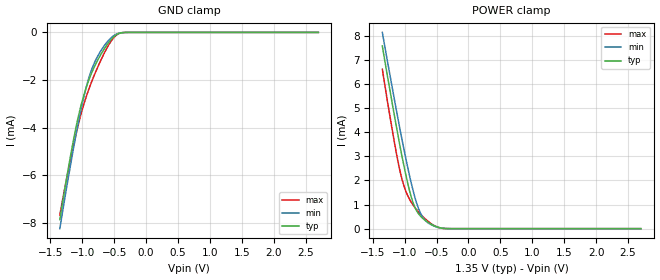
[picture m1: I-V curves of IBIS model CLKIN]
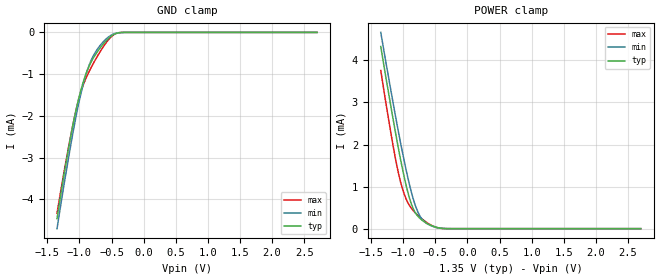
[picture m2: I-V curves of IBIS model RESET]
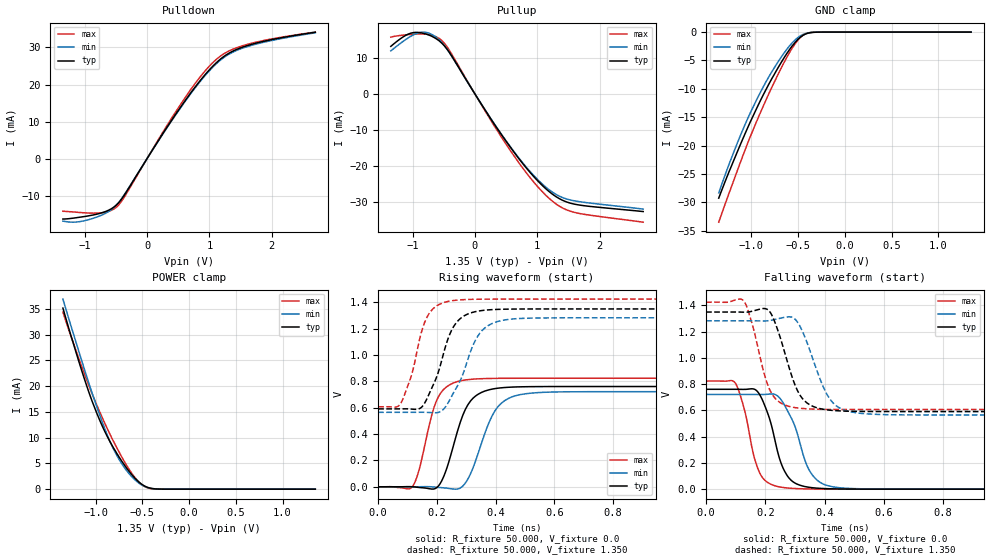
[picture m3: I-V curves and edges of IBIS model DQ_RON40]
| This Model is valid for Temperature Range -40C<=Tc<=95C
| Valid for DDR3-1600/1866 operation
| Part Number   VDD/VDDQ   Architecture   Package
| SCB13H8G162DF_DIE   1.35V/1.35V   512Mx8   Bare Die
[IBIS ver]  5.1
[File name] scb13h8g162df_die.ibs
[File Rev]  1.10
[Date]   2024-08-01
[Source]   Simulation of a silicon level SPICE model
[Notes]   Revision History:
   Rev 1.00: 2024-05-20
   - Initial release
   Rev 1.10: 2024-08-01
   - add bare die model
[Disclaimer]  The IBIS models are for modeling purpose only and are
   subject to change without any notice. UniIC is not
   responsible for any problems the models may cause.
[Copyright] Copyright 2024 UniIC Semiconductors Corp. All rights reserved
| COMPONENT: SCB13H8G162DF_DIE (Bare Die)
[Component]   SCB13H8G162DF_DIE
[Manufacturer]  UniIC Semiconductors Corp.
[Package]
|   typ   min   max
R_pkg   0.001m   0.001m   0.001m
L_pkg   0.001nH   0.001nH   0.001nH
C_pkg   0.001pF   0.001pF   0.001pF
[Pin]   signal_name   model_name   R_pin   L_pin   C_pin
1   VSS   GND
2   VDDP   POWER
3   VDD   POWER
4   RESETB   RESET
5   VDD   POWER
6   A13   INPUT
7   A9   INPUT
8   A7   INPUT
9   A2   INPUT
10   A5   INPUT
11   A0   INPUT
12   A3   INPUT
13   BA2   INPUT
14   BA0   INPUT
15   VSS   GND
16   VDD   POWER
17   WEB   INPUT
18   CSB   INPUT
19   CASB   INPUT
20   ODT   ODT
21   RASB   INPUT
22   VDD   POWER
23   VSS   GND
24   VREFDQ   POWER
25   VSS   GND
26   DQL7   DQ
27   VDDQ   POWER
28   VSS   GND
29   DQL5   DQ
30   VDDQ   POWER
31   DQL3   DQ
32   VSS   GND
33   DQL1   DQ
34   VSS   GND
35   DML   DM
36   VSS   GND
37   VDD   POWER
38   VSS   GND
39   VSS   GND
40   VDD   POWER
41   VSS   GND
42   A14   INPUT
43   A11   INPUT
44   A8   INPUT
45   A1   INPUT
46   A6   INPUT
47   A4   INPUT
48   VSS   GND
49   VDD   POWER
50   A12   INPUT
51   A15   INPUT
52   BA1   INPUT
53   ZQ   INPUT
54   VREFCA   POWER
55   A10   INPUT
56   CKE   INPUT
57   CKB   CLKIN
58   CK   CLKIN
59   VSS   GND
60   VDD   POWER
61   DQL4   DQ
62   VDDQ   POWER
63   DQL6   DQ
64   VSS   GND
65   DQSLB   DQS
66   DQSL   DQS
67   DQL2   DQ
68   VDDQ   POWER
69   DQL0   DQ
70   VDDQ   POWER
71   VDD   POWER
72   VDDQ   POWER
|**********************DIFF PIN*********************************************
[Diff_pin]   inv_pin   vdiff   tdelay_typ   tdelay_min   tdelay_max
   58   57   0.320V   0ns   NA   NA
   66   65   0.320V   0ns   NA   NA
|   Model Selector
[Model Selector] DQ
DQ_RON34   DQ  With 34ohm driving & Without ODT
DQ_RON40   DQ  With 40ohm driving & Without ODT
DQ_ODTOFF   DQ  Input with ODT OFF
DQ_ODT20   DQ  Input with 20ohm ODT
DQ_ODT30   DQ  Input with 30ohm ODT
DQ_ODT40   DQ  Input with 40ohm ODT
DQ_ODT60   DQ  Input with 60ohm ODT
DQ_ODT120   DQ  Input with 120ohm ODT
[Model Selector] DQS
DQS_RON34   DQS with 34ohm driving & Without ODT
DQS_RON40   DQS with 40ohm driving & Without ODT
DQS_ODTOFF   DQS Input with ODT OFF
DQS_ODT20   DQS Input with 20ohm ODT
DQS_ODT30   DQS Input with 30ohm ODT
DQS_ODT40   DQS Input with 40ohm ODT
DQS_ODT60   DQS Input with 60ohm ODT
DQS_ODT120   DQS Input with 120ohm ODT
[Model Selector] DM
DM_ODTOFF   DM Input with ODT OFF
DM_ODT20   DM Input with 20ohm ODT
DM_ODT30   DM Input with 30ohm ODT
DM_ODT40   DM Input with 40ohm ODT
DM_ODT60   DM Input with 60ohm ODT
DM_ODT120   DM Input with 120ohm ODT
| Models and submodels in the file (41): CLKIN (Input), INPUT (Input), RESET (Input), ODT (Input), DQ_RON34 (I/O), DQ_RON40 (I/O), DQ_ODTOFF (Input), DQ_ODT20 (Input), DQ_ODT30 (Input), DQ_ODT40 (Input), DQ_ODT60 (Input), DQ_ODT120 (Input), DQS_RON34 (I/O), DQS_RON40 (I/O), DQS_ODTOFF (Input), DQS_ODT20 (Input), DQS_ODT30 (Input), DQS_ODT40 (Input), DQS_ODT60 (Input), DQS_ODT120 (Input), DM_ODTOFF (Input), DM_ODT20 (Input), DM_ODT30 (Input), DM_ODT40 (Input), DM_ODT60 (Input), DM_ODT120 (Input), DQ_20ohm_ODT (Dynamic_clamp), DQ_30ohm_ODT (Dynamic_clamp), DQ_40ohm_ODT (Dynamic_clamp), DQ_60ohm_ODT (Dynamic_clamp), DQ_120ohm_ODT (Dynamic_clamp), DQS_20ohm_ODT (Dynamic_clamp), DQS_30ohm_ODT (Dynamic_clamp), DQS_40ohm_ODT (Dynamic_clamp), DQS_60ohm_ODT (Dynamic_clamp), DQS_120ohm_ODT (Dynamic_clamp), DM_20ohm_ODT (Dynamic_clamp), DM_30ohm_ODT (Dynamic_clamp), DM_40ohm_ODT (Dynamic_clamp), DM_60ohm_ODT (Dynamic_clamp), DM_120ohm_ODT (Dynamic_clamp)
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|   Model CLKIN
[Model] CLKIN
Model_type Input
Polarity   Non-Inverting
Enable   Active-High
Vinl =  0.550V
Vinh =  0.800V
C_comp   0.645pF   0.638pF   0.647pF
C_comp_power_clamp   0.143pF   0.139pF   0.145pF
C_comp_gnd_clamp   0.502pF   0.500pF   0.502pF
[Temperature Range]   45.000   95.000   -40.000
[Voltage Range]   1.350V   1.283V   1.425V
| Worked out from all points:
|   GND clamp passes 1 mA (typ) near -0.72 V on its own axis
|   POWER clamp passes 1 mA (typ) near -0.86 V on its own axis
[GND_clamp]
|Voltage   I(typ)   I(min)   I(max)
-1.35V    -7.873mA   -8.253mA   -7.683mA
-1.238V   -6.036mA   -6.436mA   -6.079mA
-1.125V   -4.374mA   -4.714mA   -4.633mA
-1.013V   -3.021mA   -3.17mA    -3.382mA
-928mV    -2.251mA   -2.219mA   -2.636mA
-844mV    -1.655mA   -1.511mA   -2.025mA
-759mV    -1.181mA   -1.013mA   -1.48mA
-619mV    -551.5uA   -436.8uA   -691.9uA
-506mV    -188.5uA   -137.9uA   -224uA
-422mV    -44.43uA   -32.03uA   -42.35uA
-338mV    -5.118uA   -4.402uA   -2.782uA
2.7V      0A         0A         0A
[POWER_clamp]
|Voltage   I(typ)   I(min)   I(max)
-1.35V    7.585mA    8.149mA    6.621mA
-1.153V   4.58mA     5.252mA    3.47mA
-1.097V   3.766mA    4.457mA    2.689mA
-1.041V   2.988mA    3.686mA    2.041mA
-984mV    2.262mA    2.946mA    1.57mA
-928mV    1.619mA    2.251mA    1.24mA
-844mV    908.9uA    1.339mA    892.5uA
-759mV    541.8uA    679.8uA    624.6uA
-647mV    285.5uA    268.6uA    333.7uA
-506mV    86.29uA    73.86uA    85.78uA
-366mV    7.504uA    7.144uA    3.873uA
2.7V      0A         0A         0A
|   Model RESET
[Model] RESET
Model_type Input
Polarity   Non-Inverting
Enable   Active-High
Vinl =  0.270V
Vinh =  1.080V
C_comp   0.551pF   0.542pF   0.555pF
C_comp_power_clamp   0.114pF   0.109pF   0.116pF
C_comp_gnd_clamp   0.437pF   0.433pF   0.439pF
[Temperature Range]   45.000   95.000   -40.000
[Voltage Range]   1.350V   1.283V   1.425V
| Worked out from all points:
|   GND clamp passes 1 mA (typ) near -0.90 V on its own axis
|   POWER clamp passes 1 mA (typ) near -0.95 V on its own axis
[GND_clamp]
|Voltage   I(typ)   I(min)   I(max)
-1.35V    -4.459mA   -4.699mA   -4.332mA
-1.238V   -3.374mA   -3.617mA   -3.314mA
-1.097V   -2.175mA   -2.364mA   -2.167mA
-1.013V   -1.587mA   -1.704mA   -1.607mA
-928mV    -1.122mA   -1.16mA    -1.204mA
-872mV    -885.7uA   -877.9uA   -1.006mA
-788mV    -622.5uA   -570.5uA   -752.1uA
-675mV    -364.9uA   -305.9uA   -453.3uA
-563mV    -165.4uA   -128.1uA   -202.9uA
-450mV    -38.09uA   -27.42uA   -40.32uA
-338mV    -2.553uA   -2.201uA   -1.39uA
2.7V      0A         0A         0A
[POWER_clamp]
|Voltage   I(typ)   I(min)   I(max)
-1.35V    4.331mA    4.667mA    3.761mA
-1.266V   3.557mA    3.918mA    2.946mA
-1.153V   2.561mA    2.949mA    1.928mA
-1.069V   1.859mA    2.255mA    1.281mA
-1.012V   1.425mA    1.815mA    950.8uA
-928mV    862.1uA    1.21mA     617uA
-844mV    472.4uA    705.3uA    428.3uA
-759mV    272.3uA    354.4uA    298.8uA
-647mV    139.8uA    137.3uA    161uA
-506mV    42.4uA     36.88uA    42.07uA
-366mV    3.748uA    3.583uA    1.942uA
2.7V      0A         0A         0A
|   Model DQ_RON40
[Model] DQ_RON40
Model_type I/O
Polarity   Non-Inverting
Enable   Active-High
Vinl =  0.545V
Vinh =  0.805V
Vmeas =  0.675V
Cref =  0.0F
Rref =  50.000
Vref =  0.675V
C_comp   0.962pF   0.943pF   0.974pF
C_comp_pullup   0.232pF   0.222pF   0.238pF
C_comp_pulldown   0.730pF   0.721pF   0.736pF
[Temperature Range]   45.000   95.000   -40.000
[Voltage Range]   1.350V   1.283V   1.425V
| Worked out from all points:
|   slope of the pulldown table from 0 to 0.203 V, typ, clamps not added: 37.6 ohm
|   slope of the pullup table from 0 to 0.203 V, typ, clamps not added: 36.9 ohm
|   GND clamp passes 1 mA (typ) near -0.48 V on its own axis
|   POWER clamp passes 1 mA (typ) near -0.51 V on its own axis
|   rising waveform, R_fixture 50.000, V_fixture 0.0: 20-80 % time 66.8ps typ, 75.1ps min, 56.5ps max; typ from 0 V to 0.761 V
|   rising waveform, R_fixture 50.000, V_fixture 1.350: 20-80 % time 71.2ps typ, 82.6ps min, 59.3ps max; typ from 0.591 V to 1.35 V
|   falling waveform, R_fixture 50.000, V_fixture 0.0: 20-80 % time 58.8ps typ, 68.9ps min, 50.6ps max; typ from 0.761 V to 0 V
|   falling waveform, R_fixture 50.000, V_fixture 1.350: 20-80 % time 66.4ps typ, 74.8ps min, 57.3ps max; typ from 1.35 V to 0.591 V
[Pulldown]
|Voltage   I(typ)   I(min)   I(max)
-1.35V    -16.29mA   -16.85mA   -14.19mA
-1.145V   -15.96mA   -17.11mA   -14.43mA
-900mV    -15.31mA   -16.28mA   -14.69mA
-655mV    -14.19mA   -14.64mA   -14.39mA
-491mV    -12.5mA    -12.53mA   -13.09mA
-368mV    -9.933mA   -9.803mA   -10.47mA
286mV     7.58mA     7.47mA     8.003mA
695mV     17.6mA     17.38mA    18.5mA
982mV     23.62mA    23.37mA    24.62mA
1.227V    27.49mA    27.22mA    28.23mA
1.718V    31.02mA    30.76mA    31.29mA
2.7V      34.1mA     33.95mA    34.14mA
[Pullup]
|Voltage   I(typ)   I(min)   I(max)
-1.35V    13.16mA    11.91mA    15.72mA
-1.105V   16.28mA    15.14mA    16.36mA
-900mV    17.01mA    16.95mA    16.6mA
-736mV    16.29mA    16.81mA    16.44mA
-573mV    14.68mA    14.95mA    15.34mA
-409mV    11.44mA    11.45mA    12.06mA
245mV     -6.628mA   -6.587mA   -7.019mA
695mV     -17.68mA   -17.5mA    -18.8mA
1.023V    -24.32mA   -23.97mA   -25.96mA
1.309V    -28.49mA   -27.86mA   -30.52mA
1.636V    -30.61mA   -29.69mA   -32.92mA
2.7V      -32.53mA   -31.85mA   -35.47mA
[GND_clamp]
|Voltage   I(typ)   I(min)   I(max)
-1.35V    -29.26mA   -28.34mA   -33.49mA
-1.238V   -24.53mA   -23.21mA   -28.3mA
-1.097V   -18.99mA   -17.39mA   -22.02mA
-1.013V   -15.85mA   -14.25mA   -18.44mA
-872mV    -11.01mA   -9.597mA   -12.98mA
-731mV    -6.729mA   -5.642mA   -7.982mA
-619mV    -3.711mA   -2.975mA   -4.366mA
-534mV    -1.839mA   -1.403mA   -2.088mA
-450mV    -579.7uA   -428.9uA   -569.3uA
-394mV    -185.5uA   -144.2uA   -144.2uA
-281mV    -9.318uA   -9.811uA   -3.103uA
1.35V     0A         0A         0A
[POWER_clamp]
|Voltage   I(typ)   I(min)   I(max)
-1.35V    35.16mA    36.91mA    34.39mA
-1.181V   24.89mA    26.83mA    25.44mA
-1.069V   18.67mA    20.39mA    19.96mA
-956mV    13.38mA    14.37mA    15mA
-872mV    10.11mA    10.36mA    11.63mA
-787mV    7.358mA    7.025mA    8.526mA
-703mV    4.977mA    4.465mA    5.69mA
-619mV    2.933mA    2.534mA    3.219mA
-534mV    1.338mA    1.137mA    1.316mA
-450mV    385.5uA    342uA      284.3uA
-366mV    62.9uA     66.43uA    27.04uA
1.35V     0A         0A         9.135nA
[Ramp]
| variable   typ   min   max
dV/dt_r   0.457/67.068p   0.433/75.437p   0.494/56.454p
dV/dt_f   0.455/66.331p   0.431/74.640p   0.491/58.220p
R_load = 50.000
[Rising Waveform]
R_fixture= 50.000
V_fixture= 0.0
V_fixture_min= 0.0
V_fixture_max= 0.0
|time   V(typ)   V(min)   V(max)
0s        104.4nV    279.9nV    10.03uV
119ps     -364.1uV   -73.9uV    8.881mV
203ps     464.6uV    -4.308mV   673.4mV
232ps     129.5mV    -10.12mV   756.8mV
280ps     492mV      -8.598mV   804mV
325ps     676mV      154.5mV    817.3mV
378ps     736.2mV    489.8mV    822.1mV
411ps     749.3mV    615.4mV    823.2mV
543ps     760.4mV    714.7mV    824mV
5ns       761.1mV    722mV      824mV
[Rising Waveform]
R_fixture= 50.000
V_fixture= 1.350
V_fixture_min= 1.283
V_fixture_max= 1.425
|time   V(typ)   V(min)   V(max)
0s        591.3mV    565.2mV    607mV
79ps      591.3mV    565.2mV    642mV
114ps     589.6mV    565.2mV    851.1mV
151ps     611.7mV    565.6mV    1.201V
218ps     972.9mV    578.8mV    1.394V
248ps     1.178V     677.4mV    1.411V
280ps     1.277V     808.1mV    1.419V
354ps     1.338V     1.186V     1.424V
488ps     1.349V     1.278V     1.425V
5ns       1.35V      1.283V     1.425V
[Falling Waveform]
R_fixture= 50.000
V_fixture= 0.0
V_fixture_min= 0.0
V_fixture_max= 0.0
|time   V(typ)   V(min)   V(max)
0s        761.1mV    722mV      824mV
101ps     761.2mV    722mV      799.9mV
130ps     760.5mV    722mV      600.8mV
174ps     742.8mV    721.6mV    161.5mV
213ps     546.3mV    724.5mV    44.51mV
239ps     309mV      714.3mV    21.87mV
285ps     72.74mV    554.5mV    7.154mV
361ps     10.55mV    102.2mV    1.212mV
473ps     917.5uV    6.806mV    89.78uV
5ns       106.7nV    279.9nV    9.968uV
[Falling Waveform]
R_fixture= 50.000
V_fixture= 1.350
V_fixture_min= 1.283
V_fixture_max= 1.425
|time   V(typ)   V(min)   V(max)
0s        1.35V      1.283V     1.425V
128ps     1.349V     1.283V     1.432V
210ps     1.365V     1.284V     785mV
239ps     1.232V     1.297V     679.3mV
291ps     852mV      1.31V      625.4mV
332ps     674mV      1.169V     613.8mV
394ps     609.7mV    788.5mV    608.5mV
428ps     600mV      659.2mV    607.7mV
546ps     592mV      573.5mV    607mV
5ns       591.3mV    565.2mV    607mV
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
